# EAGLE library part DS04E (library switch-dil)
DIL/CODE SWITCH
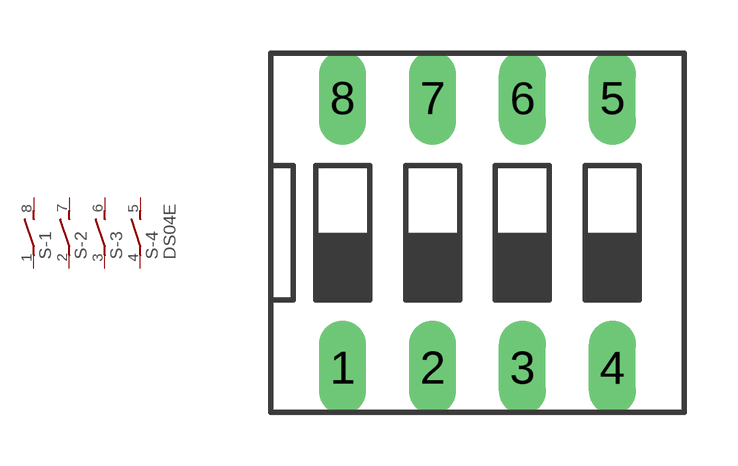
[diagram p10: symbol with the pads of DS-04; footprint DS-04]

Designator prefix S; gates -1=S -2=S -3=S -4=S+V

## DS04E (OC_FARNELL: unknown; OC_NEWARK: unknown)  [DS-04]
1  -1:1  pas
2  -2:1  pas
3  -3:1  pas
4  -4:1  pas
5  -4:2  pas
6  -3:2  pas
7  -2:2  pas
8  -1:2  pas

## Footprint DS-04 (pad centres in mm)
DIL/CODE SWITCH Mors distributor Buerklin, 17G554
drill 0.813 long: 1 -3.81,-3.81; 2 -1.27,-3.81; 3 1.27,-3.81; 4 3.81,-3.81; 5 3.81,3.81; 6 1.27,3.81; 7 -1.27,3.81; 8 -3.81,3.81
